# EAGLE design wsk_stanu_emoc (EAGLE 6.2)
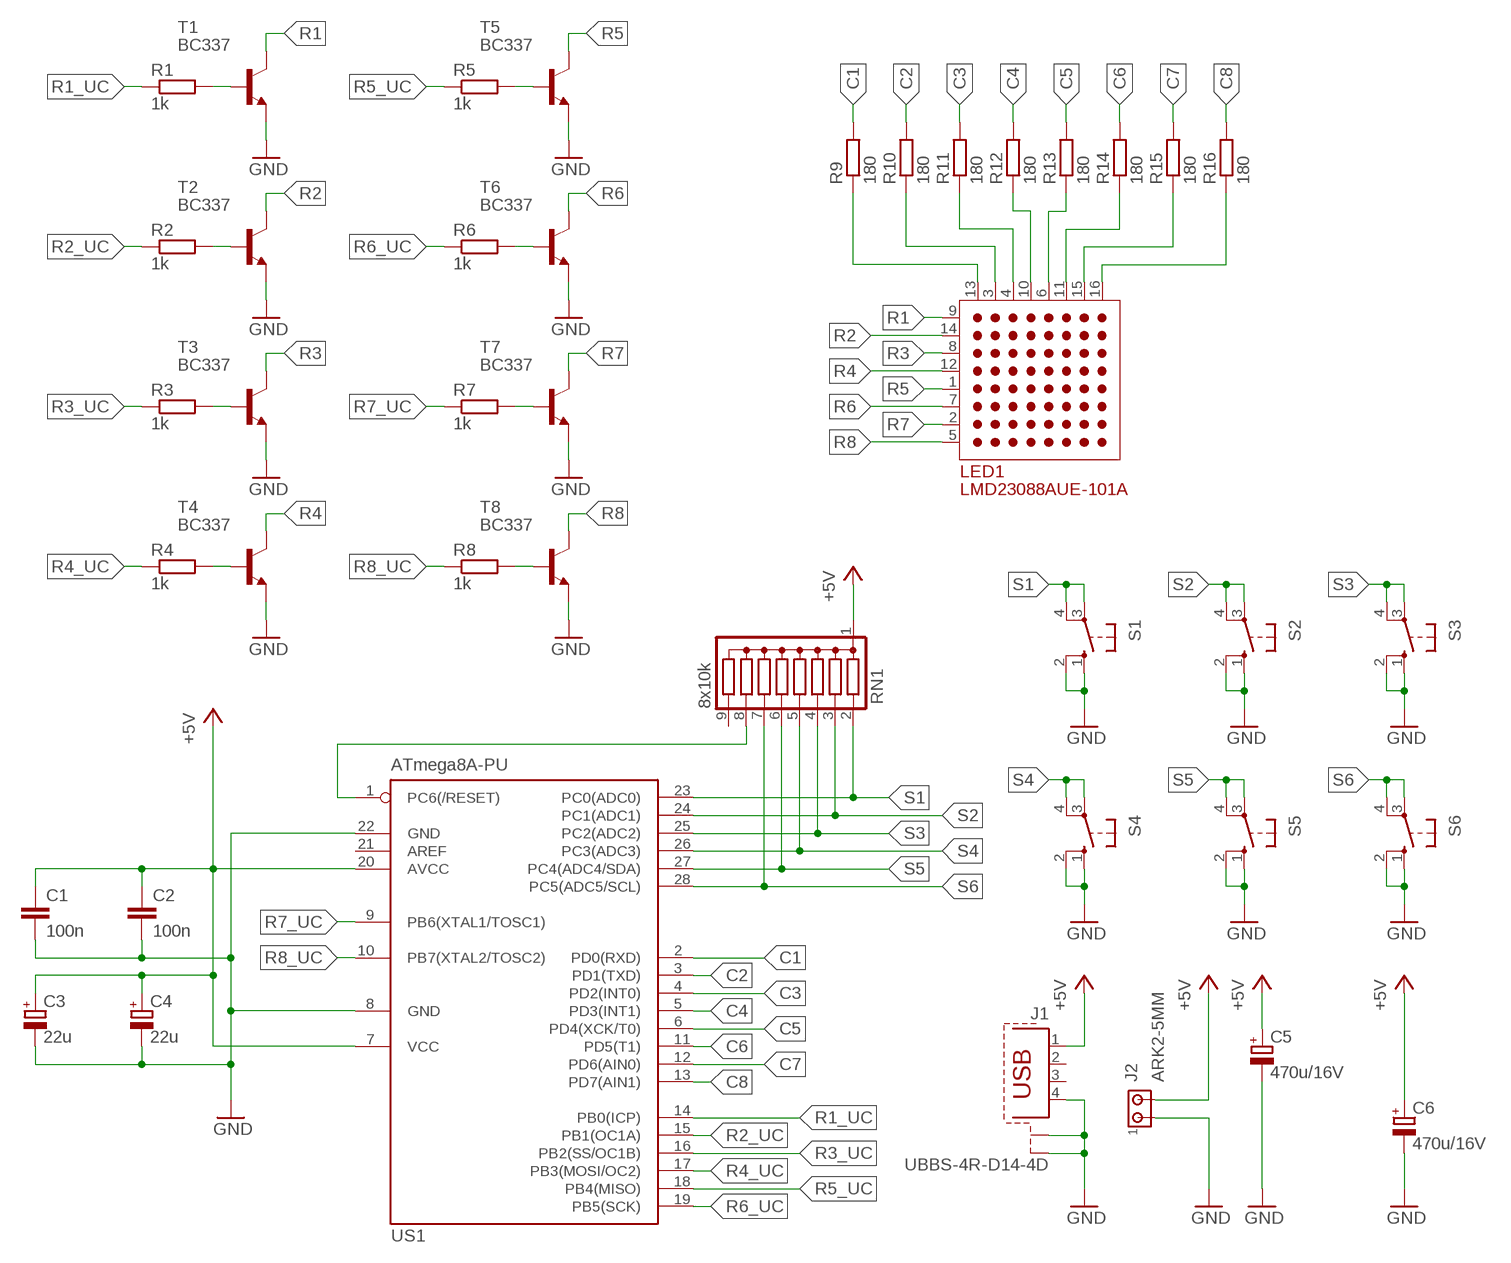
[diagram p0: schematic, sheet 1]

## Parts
C1  100n  C-EU050-025X075  [C050-025X075]
C2  100n  C-EU050-025X075  [C050-025X075]
C3  22u  CPOL-EUE2.5-6  [E2,5-6]
C4  22u  CPOL-EUE2.5-6  [E2,5-6]
C5  470u/16V  CPOL-EUE3.5-8  [E3,5-8]
C6  470u/16V  CPOL-EUE3.5-8  [E3,5-8]
J1  UBBS-4R-D14-4D  USB_B_PION_UBBS-4R-D14-4D  [USB_B_PION_UBBS-4R-D14-4D]
J2  ARK2-5MM  [2PIN-5MM]
LED1  LMD23088AUE-101A  KWM-50881  [KWM-50881]
R1  1k  R-EU_0207/7  [0207/7]
R2  1k  R-EU_0207/7  [0207/7]
R3  1k  R-EU_0207/7  [0207/7]
R4  1k  R-EU_0207/7  [0207/7]
R5  1k  R-EU_0207/7  [0207/7]
R6  1k  R-EU_0207/7  [0207/7]
R7  1k  R-EU_0207/7  [0207/7]
R8  1k  R-EU_0207/7  [0207/7]
R9  180  R-EU_0207/7  [0207/7]
R10  180  R-EU_0207/7  [0207/7]
R11  180  R-EU_0207/7  [0207/7]
R12  180  R-EU_0207/7  [0207/7]
R13  180  R-EU_0207/7  [0207/7]
R14  180  R-EU_0207/7  [0207/7]
R15  180  R-EU_0207/7  [0207/7]
R16  180  R-EU_0207/7  [0207/7]
RN1  8x10k  DRAB_REZ_1X8-SIL9  [RN-9]
S1  10-XX  [B3F-10XX]
S2  10-XX  [B3F-10XX]
S3  10-XX  [B3F-10XX]
S4  10-XX  [B3F-10XX]
S5  10-XX  [B3F-10XX]
S6  10-XX  [B3F-10XX]
T1  BC337  BC546A  [TO92-EBC]
T2  BC337  BC546A  [TO92-EBC]
T3  BC337  BC546A  [TO92-EBC]
T4  BC337  BC546A  [TO92-EBC]
T5  BC337  BC546A  [TO92-EBC]
T6  BC337  BC546A  [TO92-EBC]
T7  BC337  BC546A  [TO92-EBC]
T8  BC337  BC546A  [TO92-EBC]
US1  ATmega8A-PU  MEGA8-P  [DIL28-3]

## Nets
+5V: C1.1 C2.1 C3.+ C4.+ C5.+ C6.+ J1.1 J2.P$2 RN1.1(C) US1.7(VCC) US1.20(AVCC)
C1: R9.2 US1.2(PD0(RXD))
C2: R10.2 US1.3(PD1(TXD))
C3: R11.2 US1.4(PD2(INT0))
C4: R12.2 US1.5(PD3(INT1))
C5: R13.2 US1.6(PD4(XCK/T0))
C6: R14.2 US1.11(PD5(T1))
C7: R15.2 US1.12(PD6(AIN0))
C8: R16.2 US1.13(PD7(AIN1))
GND: C1.2 C2.2 C3.- C4.- C5.- C6.- J1.4 J1.GND1(S1) J1.GND2(S2) J2.P$1 S1.1(S) S1.2(S1) S2.1(S) S2.2(S1) S3.1(S) S3.2(S1) S4.1(S) S4.2(S1) S5.1(S) S5.2(S1) S6.1(S) S6.2(S1) T1.E T2.E T3.E T4.E T5.E T6.E T7.E T8.E US1.8(GND) US1.22(GND)
N$1: RN1.8 US1.1(PC6(/RESET))
N$2: LED1.10(C4) R12.1
N$3: LED1.6(C5) R13.1
N$4: LED1.4(C3) R11.1
N$5: LED1.3(C2) R10.1
N$6: LED1.13(C1) R9.1
N$7: LED1.11(C6) R14.1
N$8: LED1.15(C7) R15.1
N$9: R1.2 T1.B
N$10: LED1.16(C8) R16.1
N$12: R2.2 T2.B
N$13: R3.2 T3.B
N$14: R4.2 T4.B
N$15: R5.2 T5.B
N$16: R6.2 T6.B
N$17: R7.2 T7.B
N$18: R8.2 T8.B
R1: LED1.9(R1) T1.C
R1_UC: R1.1 US1.14(PB0(ICP))
R2: LED1.14(R2) T2.C
R2_UC: R2.1 US1.15(PB1(OC1A))
R3: LED1.8(R3) T3.C
R3_UC: R3.1 US1.16(PB2(SS/OC1B))
R4: LED1.12(R4) T4.C
R4_UC: R4.1 US1.17(PB3(MOSI/OC2))
R5: LED1.1(R5) T5.C
R5_UC: R5.1 US1.18(PB4(MISO))
R6: LED1.7(R6) T6.C
R6_UC: R6.1 US1.19(PB5(SCK))
R7: LED1.2(R7) T7.C
R7_UC: R7.1 US1.9(PB6(XTAL1/TOSC1))
R8: LED1.5(R8) T8.C
R8_UC: R8.1 US1.10(PB7(XTAL2/TOSC2))
S1: RN1.2 S1.3(P) S1.4(P1) US1.23(PC0(ADC0))
S2: RN1.3 S2.3(P) S2.4(P1) US1.24(PC1(ADC1))
S3: RN1.4 S3.3(P) S3.4(P1) US1.25(PC2(ADC2))
S4: RN1.5 S4.3(P) S4.4(P1) US1.26(PC3(ADC3))
S5: RN1.6 S5.3(P) S5.4(P1) US1.27(PC4(ADC4/SDA))
S6: RN1.7 S6.3(P) S6.4(P1) US1.28(PC5(ADC5/SCL))
Unconnected: J1.2 J1.3 RN1.9 US1.21(AREF)

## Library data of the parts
C1 C2 = rcl:C-EU: CAPACITOR, European symbol
C3-C6 = rcl:CPOL-EU: POLARIZED CAPACITOR, European symbol
J1 = zlacza_futrzak:USB_B_PION_UBBS-4R-D14-4D
J2 = zlacza_futrzak:ARK2: ARK 2
LED1 = ledmatrix:KWM-50881
R1-R16 = rcl:R-EU_: RESISTOR, European symbol
RN1 = inne_futrzak:DRAB_REZ_1X8
S1-S6 = switch-omron:10-XX: OMRON SWITCH; MPN: B3F-1000; OC_FARNELL: 176432; OC_NEWARK: 36M3542
T1-T8 = transistor-npn:BC546*: NPN Transistor
US1 = atmel:MEGA8-P: MICROCONTROLLER 8 Kbytes FLASH, 1 kbytes SRAM, 512 bytes EEPROM, USART, 4-channel 10 bit ADC, 2-channel 8 bit ADC Pin compatible with Atmega48, ATMega88, ATMega168 Source: avr.lbr; OC_FARNELL: unknown; OC_NEWARK: unknown

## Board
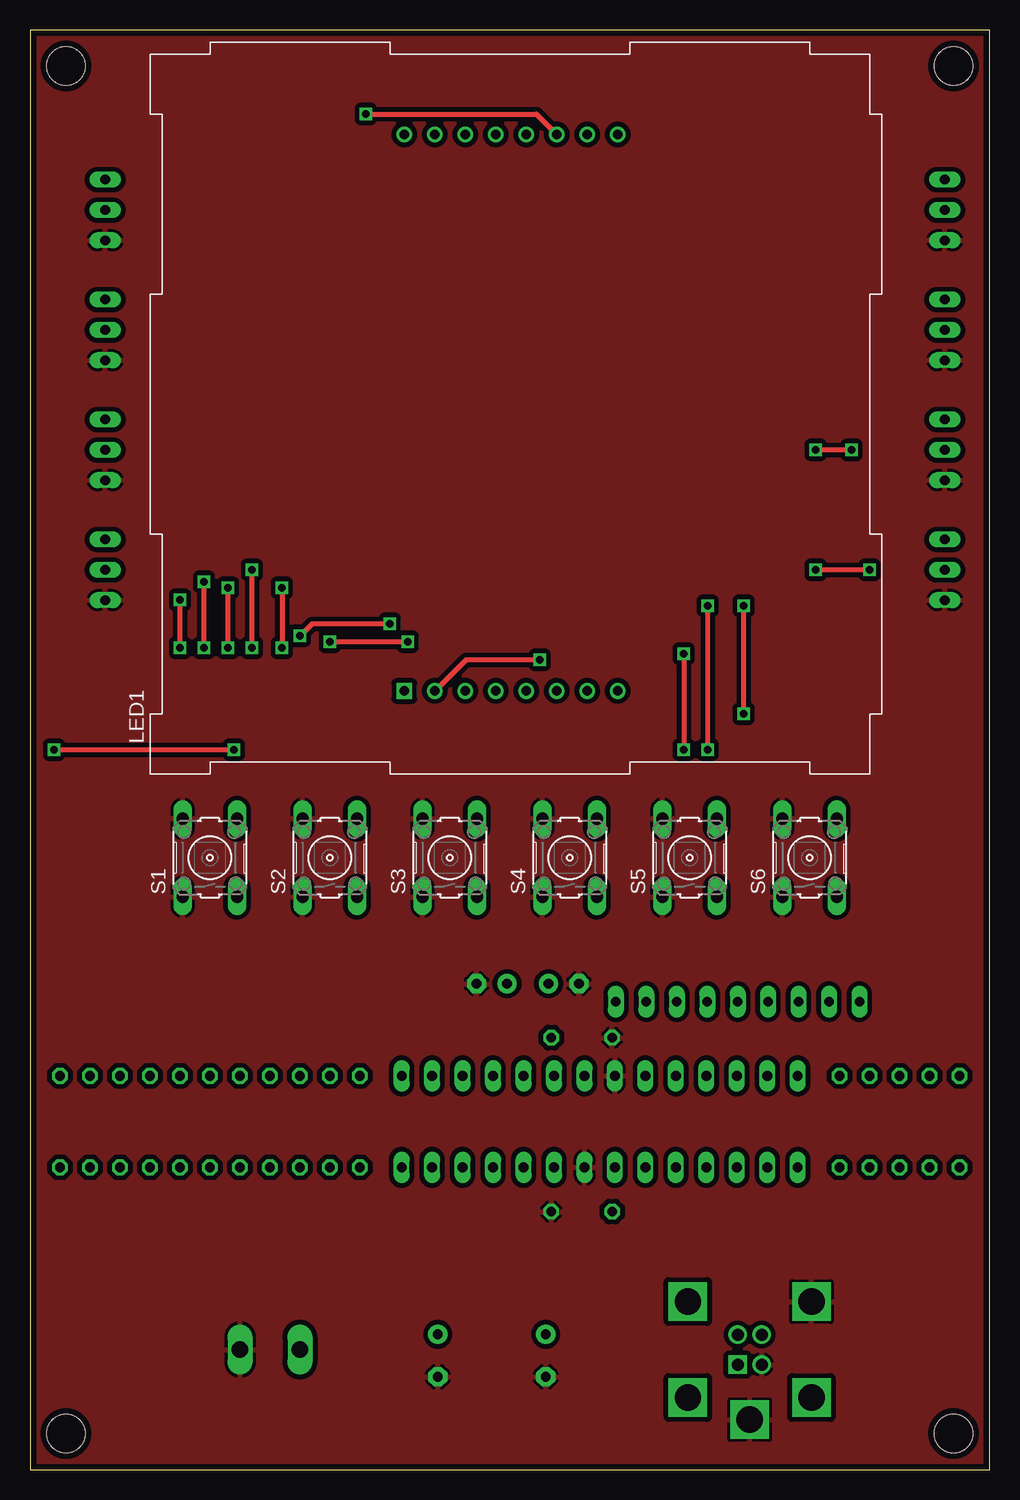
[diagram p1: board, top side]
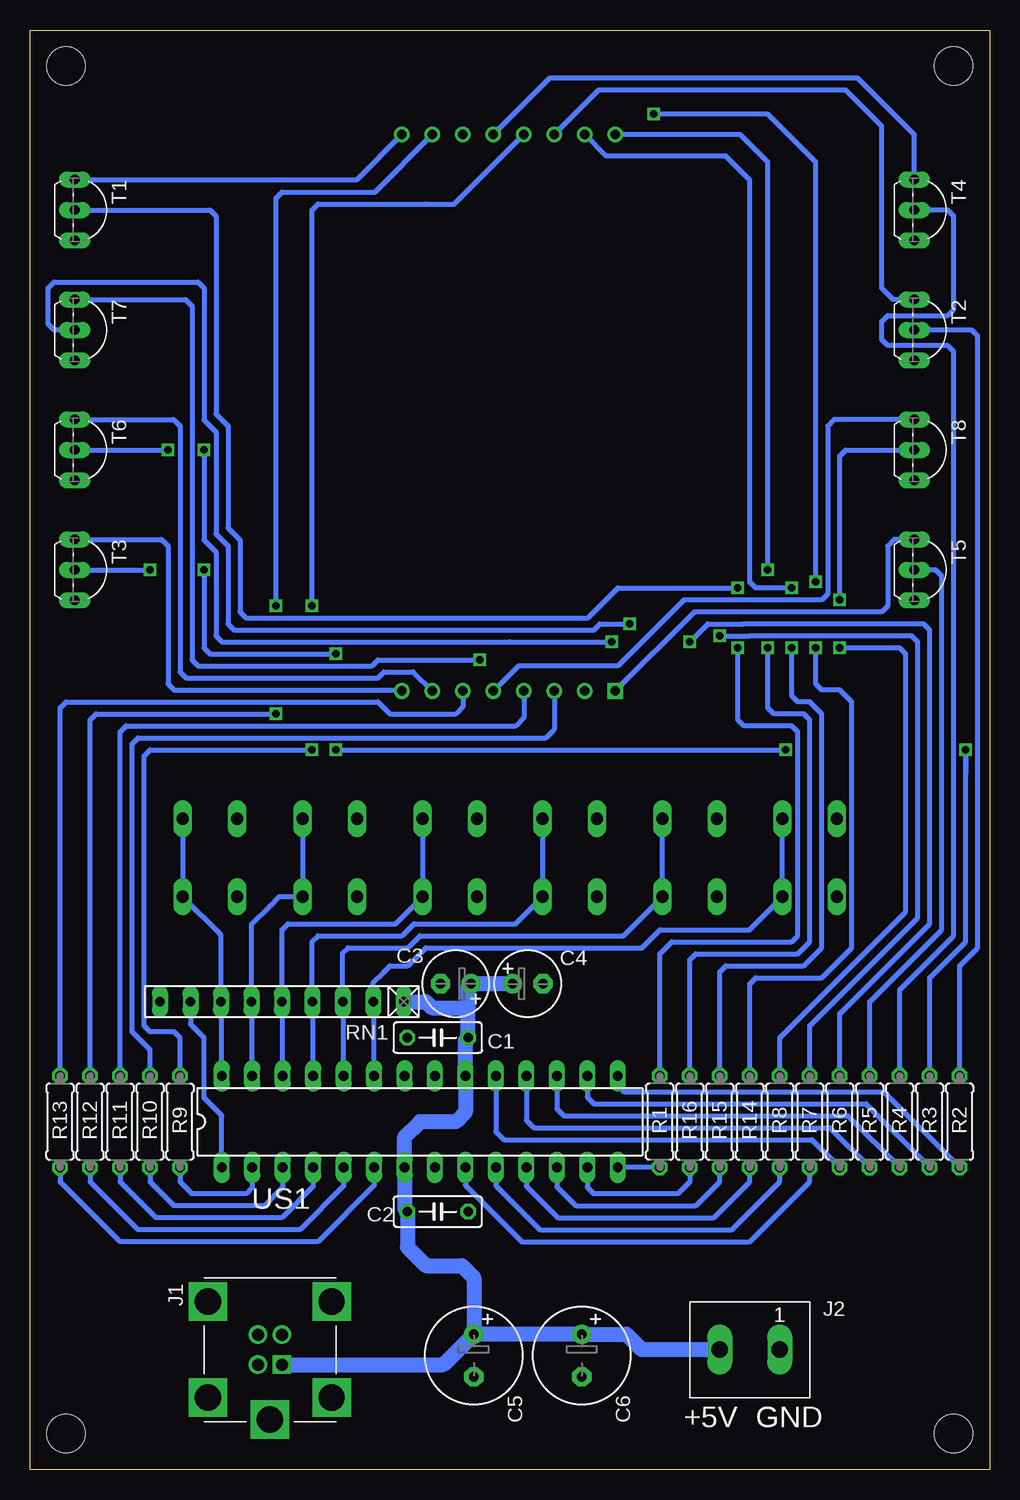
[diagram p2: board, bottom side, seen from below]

Size 80 x 120 mm. Coordinates in mm from the lower left corner, seen from the top.
Outline: 0,0 80,0 80,120 0,120 0,0
Copper layers (1*16): Top 0.035mm / dielectric 1.5mm / Bottom 0.035mm
Design rules: minimum track width 10mil, minimum drill 23mil, track to track 8mil, track to pad 8mil, pad to pad 8mil, via to via 8mil, smd to smd 8mil, copper to edge 20mil, drill to drill 8mil, minimum pad ring 10mil, minimum via ring 8mil, stop-mask expansion 4mil, vias tented up to drill 0mil, thermal gap 10mil
Holes 3.2 mm at 3,117 77,117 3,3 77,3

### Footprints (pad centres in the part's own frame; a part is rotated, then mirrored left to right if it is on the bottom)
C050-025X075 = drill 0.813 octagon: 1 -2.54,0; 2 2.54,0
E2,5-6 = drill 0.813 pad 1.6: + -1.27,0 | drill 0.813 pad 1.6 octagon: - 1.27,0
E3,5-8 = drill 0.813 pad 1.6: + -1.778,0 | drill 0.813 pad 1.6 octagon: - 1.778,0
USB_B_PION_UBBS-4R-D14-4D = drill 1 square: 1 1.25,1 | drill 1: 2 -1.25,1; 3 -1.25,-1; 4 1.25,-1 | drill 2.2 square: GND1 5.85,0; GND2 -4,-5.15; P$2 4,5.15; P$3 -4,5.15; P$5 4,-5.15
2PIN-5MM = drill 1.4 long: P$1 -2.5,0; P$2 2.5,0
KWM-50881 = drill 0.8 square: 1 21.21,6.9 | drill 0.8: 2 23.75,6.9; 3 26.29,6.9; 4 28.83,6.9; 5 31.37,6.9; 6 33.91,6.9; 7 36.45,6.9; 8 38.99,6.9; 9 38.99,53.3; 10 36.45,53.3; 11 33.91,53.3; 12 31.37,53.3; 13 28.83,53.3; 14 26.29,53.3; 15 23.75,53.3; 16 21.21,53.3
0207/7 = drill 0.813 octagon: 1 -3.81,0; 2 3.81,0
RN-9 = drill 0.813 long: 1 -10.16,0; 2 -7.62,0; 3 -5.08,0; 4 -2.54,0; 5 0,0; 6 2.54,0; 7 5.08,0; 8 7.62,0; 9 10.16,0
B3F-10XX = drill 1.016 long: 1 -3.251,2.261; 2 3.251,2.261; 3 -3.251,-2.261; 4 3.251,-2.261
TO92-EBC = drill 0.813 long: B 0,-1.27; C -2.54,-1.27; E 2.54,-1.27
DIL28-3 = drill 0.813 long: 1 -16.51,-3.81; 2 -13.97,-3.81; 3 -11.43,-3.81; 4 -8.89,-3.81; 5 -6.35,-3.81; 6 -3.81,-3.81; 7 -1.27,-3.81; 8 1.27,-3.81; 9 3.81,-3.81; 10 6.35,-3.81; 11 8.89,-3.81; 12 11.43,-3.81; 13 13.97,-3.81; 14 16.51,-3.81; 15 16.51,3.81; 16 13.97,3.81; 17 11.43,3.81; 18 8.89,3.81; 19 6.35,3.81; 20 3.81,3.81; 21 1.27,3.81; 22 -1.27,3.81; 23 -3.81,3.81; 24 -6.35,3.81; 25 -8.89,3.81; 26 -11.43,3.81; 27 -13.97,3.81; 28 -16.51,3.81

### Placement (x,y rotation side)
C1  46,36 180 bottom
C2  46,21.5 0 bottom
C3  44.5,40.5 180 bottom
C4  38.5,40.5 0 bottom
C5  43,9.5 270 bottom
C6  34,9.5 270 bottom
J1  60,10 270 bottom
J2  20,10 180 bottom
LED1  10,58 0 top
R1  27.5,29 90 bottom
R2  2.5,29 90 bottom
R3  5,29 90 bottom
R4  7.5,29 90 bottom
R5  10,29 90 bottom
R6  12.5,29 90 bottom
R7  15,29 90 bottom
R8  17.5,29 90 bottom
R9  67.5,29 270 bottom
R10  70,29 270 bottom
R11  72.5,29 270 bottom
R12  75,29 270 bottom
R13  77.5,29 270 bottom
R14  20,29 270 bottom
R15  22.5,29 270 bottom
R16  25,29 270 bottom
RN1  59,39 180 bottom
S1  15,51 90 top
S2  25,51 90 top
S3  35,51 90 top
S4  45,51 90 top
S5  55,51 90 top
S6  65,51 90 top
T1  75,105 270 bottom
T2  5,95 270 bottom
T3  75,75 270 bottom
T4  5,105 270 bottom
T5  5,75 270 bottom
T6  75,85 270 bottom
T7  75,95 270 bottom
T8  5,85 270 bottom
US1  47.5,29 0 bottom

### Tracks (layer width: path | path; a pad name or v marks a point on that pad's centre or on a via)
+5V
  Bottom 1.27: 43.46,38.5 C1.1 43.69,35.77 US1.20 43.69,29.81 44.5,29 47.5,29 48.77,27.73 US1.7 48.77,21.73 C2.1 48.54,18.54 47,17 44,17 43,16 C5.+ | 43.46,38.5 43.46,40.27 C3.+ C4.+ | RN1.1 47,39 46.5,38.5 43.46,38.5 | J1.1 45.53,8.75 C5.+ | C5.+ C6.+ 30.28,11.28 30,11 29,10 J2.P$2
C1
  Bottom 0.406: R9.2 67.5,24 66.5,23 62,23 61.47,23.53 US1.2
C2
  Bottom 0.406: R10.2 70,24 68,22 60.5,22 58.93,23.57 US1.3
C3
  Bottom 0.406: R11.2 72.5,24 69.5,21 59,21 56.39,23.61 US1.4
C4
  Bottom 0.406: R12.2 75,24 71,20 57.5,20 53.85,23.65 US1.5
C5
  Bottom 0.406: R13.2 77.5,24 72.5,19 56,19 51.31,23.69 US1.6
C6
  Bottom 0.406: US1.11 38.61,23.61 36,21 23,21 20,24 R14.2
C7
  Bottom 0.406: US1.12 36.07,23.57 34.5,22 24.5,22 22.5,24 R15.2
C8
  Bottom 0.406: R16.2 25,24 25.5,23.5 26,23 33,23 33.53,23.53 US1.13
GND
  pour Top (isolate 0.406): 0,0 80,0 80,120 0,120
N$1
  Bottom 0.406: US1.1 64.01,29.51 65.5,31 65.5,36 66.62,37.12 RN1.8
N$2  (via drill 0.6)
  Top 0.406: v59.5,63 v59.5,72
  Bottom 0.406: R12.1 75,60 75,62.5 74.5,63 v59.5,63 | v59.5,72 59.5,106 59,106.5 51.25,106.5 LED1.10
N$3
  Bottom 0.406: R13.1 77.5,59.5 77.5,63 77.5,63.5 77,64 51,64 50,63 44.5,63 43.91,63.59 LED1.6
N$4
  Bottom 0.406: R11.1 72.5,60.5 72.5,61.5 72,62 39.5,62 38.83,62.67 LED1.4
N$5
  Bottom 0.406: R10.1 70,35 71.5,36.5 71.5,60.5 71,61 37,61 36.5,61.5 36.29,61.71 LED1.3
N$6  (via drill 0.6)
  Top 0.406: v56.5,60 v56.5,72
  Bottom 0.406: R9.1 67.5,36 68,36.5 70,36.5 70.5,37 70.5,54.5 70.5,59.5 70,60 v56.5,60 | v56.5,72 56.5,105 56,105.5 47,105.5 44.63,105.5 LED1.13
N$7  (via drill 0.6)
  Top 0.406: v14.5,68.5 v14.5,74 | v28,113 42.21,113 LED1.11
  Bottom 0.406: R14.1 20,40.5 19.5,41 14,41 11.5,43.5 11.5,61.5 11.5,64 12.5,65 14,65 14.5,65.5 v14.5,68.5 | v14.5,74 14.5,109 18.5,113 v28,113
N$8  (via drill 0.6)
  Top 0.406: v16.5,68.5 v16.5,73.5
  Bottom 0.406: R15.1 22.5,41.5 22,42 15.5,42 14,43.5 14,61.5 14,63 15,64 16,64 16.5,64.5 v16.5,68.5 | v16.5,73.5 17,73.5 19,73.5 19.5,73.5 20,74 20,107.5 22,109.5 31.95,109.5 LED1.15
N$9  (via drill 0.6)
  Top 0.406: v21,73.5 v21,68.5
  Bottom 0.406: R1.2 27.5,43 26.5,44 16.5,44 16,44.5 16,61 16,61.5 16.5,62 20.5,62 21,62.5 v21,68.5 | T1.B 65,105 64.5,104.5 64.5,88 63.5,87 63.5,78.5 62.5,77.5 62.5,71.5 62,71 33.5,71 31,73.5 v21,73.5
N$10  (via drill 0.6)
  Top 0.406: v18.5,68.5 v18.5,75
  Bottom 0.406: R16.1 25,41.5 25,42.5 24.5,43 16,43 15,44 15,61.5 15,62.5 15.5,63 18,63 18.5,63.5 v18.5,68.5 | v18.5,75 18.5,109 20.8,111.3 LED1.16
N$12
  Bottom 0.406: R2.2 2.5,33 2.5,42 1,43.5 1,94.5 | 1,94.5 1.25,94.75 | 1.25,94.75 1.5,95 T2.B | 1,94.5 1.25,94.75
N$13  (via drill 0.6)
  Top 0.406: v70,75 v65.5,75 | v54.5,68 v54.5,60 | v17,60 v2,60
  Bottom 0.406: R3.2 5,33 5,41 2,44 2,58 | 2,58 v2,60 2,58 | T3.B v70,75 | v65.5,75 65.5,68.5 65,68 v54.5,68 | v54.5,60 v17,60
N$14
  Bottom 0.406: R4.2 7.5,40 3,44.5 3,89.5 3,93.2 3.5,93.7 8.5,93.7 9,94.2 9,95.7 8.5,96.2 3.5,96.2 3,96.7 3,104.5 3.5,105 T4.B
N$15
  Bottom 0.406: R5.2 10,39 4,45 4,74.5 4.5,75 T5.B
N$16  (via drill 0.6)
  Top 0.406: v68.5,85 v65.5,85 | v31.5,69 v25,69
  Bottom 0.406: R6.2 12.5,38 5,45.5 5,70 5.5,70.5 20.5,70.5 23.5,70.5 v25,69 | T6.B v68.5,85 | v65.5,85 65.5,77.5 64.5,76.5 64.5,69.5 64,69 40,69 v31.5,69
N$17  (via drill 0.6)
  Top 0.406: v30,70.5 23.5,70.5 v22.5,69.5
  Bottom 0.406: R7.2 15,37 6,46 6,69 6.5,69.5 20,69.5 v22.5,69.5 | T7.B 78,95 78.5,95.5 78.5,98.5 78,99 66,99 65.5,98.5 65.5,87.5 64.5,86.5 64.5,78 63.5,77 63.5,70.5 63,70 33,70 32.5,70.5 v30,70.5
N$18  (via drill 0.6)
  Top 0.406: v12.5,68.5 v12.5,72.5
  Bottom 0.406: R8.2 17.5,36 7,46.5 7,68 7.5,68.5 v12.5,68.5 | v12.5,72.5 12.5,84.5 12,85 T8.B
R1
  Bottom 0.406: T1.C 52.75,107.54 LED1.9
R1_UC
  Bottom 0.406: R1.1 US1.14
R2
  Bottom 0.406: T2.C 8.04,97.54 9,98.5 9,112 12,115 32.59,115 LED1.14
R2_UC
  Bottom 0.406: US1.15 30.99,31.99 30.5,31.5 8.81,31.5 R2.1
R3
  Bottom 0.406: T3.C 69.04,77.54 68.5,77 68.5,65.5 68,65 49.09,65 LED1.8
R3_UC
  Bottom 0.406: US1.16 33.53,31.03 33,30.5 10.31,30.5 R3.1
R4
  Bottom 0.406: T4.C 6.27,111.27 11,116 36.67,116 LED1.12
R4_UC
  Bottom 0.406: US1.17 36.07,30.07 35.5,29.5 11.81,29.5 R4.1
R5
  Bottom 0.406: T5.C 7.96,77.54 8.5,77 8.5,72 9,71.5 24.61,71.5 LED1.1
R5_UC
  Bottom 0.406: US1.18 38.61,29.11 38,28.5 13.31,28.5 R5.1
R6
  Bottom 0.406: T6.C 68.04,87.54 67.5,87 67.5,66.5 67,66 51,66 50.5,66.5 48.05,66.5 LED1.7
R6_UC
  Bottom 0.406: US1.19 41.15,28.15 40.5,27.5 14.81,27.5 R6.1
R7  (via drill 0.6)
  Top 0.406: v42.5,67.5 36.35,67.5 LED1.2
  Bottom 0.406: T7.C 67.04,97.54 66.5,97 66.5,67.5 66,67 51.5,67 51,67.5 v42.5,67.5
R7_UC
  Bottom 0.406: US1.9 43.69,23.69 39,19 20,19 15,24 R7.1
R8
  Bottom 0.406: T8.C 12.96,87.54 13.5,87 13.5,73 14,72.5 25.5,72.5 31,67 39.27,67 LED1.5
R8_UC
  Bottom 0.406: US1.10 41.15,23.65 37.5,20 21.5,20 17.5,24 R8.1
S1
  Bottom 0.406: US1.23 51.31,38.93 RN1.2 51.38,40.62 50.5,41.5 50,42 48.5,42 47,43.5 29,43.5 27.5,45 20.01,45 S1.3 S1.4
S2
  Bottom 0.406: US1.24 53.85,38.93 RN1.3 53.92,43.08 53.5,43.5 48.5,43.5 47.5,44.5 30.51,44.5 S2.3 S2.4
S3
  Bottom 0.406: US1.25 56.39,38.93 RN1.4 56.46,44.04 56,44.5 49,44.5 48,45.5 39.51,45.5 S3.3 S3.4
S4
  Bottom 0.406: US1.26 58.93,38.93 RN1.5 59,45 58.5,45.5 49.51,45.5 S4.3 S4.4
S5
  Bottom 0.406: US1.27 61.47,38.93 RN1.6 61.54,45.46 60,47 59.25,47.75 S5.3 S5.4
S6
  Bottom 0.406: US1.28 64.01,38.93 RN1.7 64.08,44.57 S6.3 S6.4

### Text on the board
bPlace: GND | +5V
